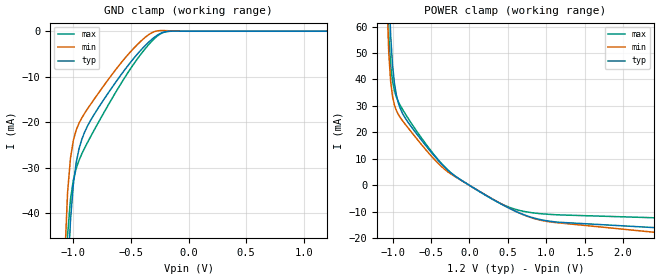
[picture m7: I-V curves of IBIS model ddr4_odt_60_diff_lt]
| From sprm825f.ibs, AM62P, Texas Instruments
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|   Model ddr4_odt_60_diff_lt
[Model] ddr4_odt_60_diff_lt
Model_type Input
Polarity   Non-Inverting
Enable   Active-High
Vinl =  0.700V
Vinh =  0.900V
C_comp   2.403pF   2.224pF   2.539pF
[Model Spec]
Vinh   0.900V   0.820V   0.980V
Vinl   0.700V   0.620V   0.780V
[Temperature Range]   25.000   -40.000   -40.000
[Voltage Range]   1.200V   1.140V   1.260V
[C Comp Corner]
C_comp   2.403pF   2.224pF   2.539pF
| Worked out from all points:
|   GND clamp passes 1 mA (typ) near -0.28 V on its own axis
|   POWER clamp passes 1 mA (typ) near -0.06 V on its own axis
[GND_clamp]
|Voltage   I(typ)   I(min)   I(max)
-1.2V     -388.2mA   -352.6mA   -364.4mA
-1.075V   -77.92mA   -50.35mA   -60.12mA
-1.05V    -55.4mA    -35.49mA   -44.9mA
-1.025V   -41.74mA   -27.93mA   -37mA
-1V       -33.68mA   -23.99mA   -32.73mA
-975mV    -28.85mA   -21.71mA   -30.14mA
-950mV    -25.78mA   -20.17mA   -28.32mA
-900mV    -22.05mA   -17.95mA   -25.56mA
-775mV    -16.53mA   -13.35mA   -19.7mA
-350mV    -2.491mA   -816.8uA   -3.051mA
-175mV    -21.61uA   107.5uA    -25.48uA
1.2V      0A         0A         0A
[POWER_clamp]
|Voltage   I(typ)   I(min)   I(max)
-1.2V     598.1mA    616mA      625.7mA
-1.075V   109.8mA    73.33mA    80.44mA
-1.05V    76.96mA    50.73mA    57.36mA
-1.025V   57.16mA    39.42mA    45.6mA
-1V       45.49mA    33.6mA     39.37mA
-975mV    38.51mA    30.33mA    35.74mA
-925mV    31.21mA    26.8mA     31.63mA
-625mV    17.14mA    15.47mA    17.96mA
-175mV    3.236mA    3.1mA      3.281mA
425mV     -7.246mA   -7.182mA   -7.141mA
850mV     -12.46mA   -12.63mA   -10.5mA
2.4V      -15.99mA   -17.74mA   -12.27mA
